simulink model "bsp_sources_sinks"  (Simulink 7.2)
settings: Solver=VariableStepDiscrete  StartTime=0.0  StopTime=1000.0  FixedStep=0.1  MaxStep=2.0  RelTol=1e-3
libraries: simulink x2

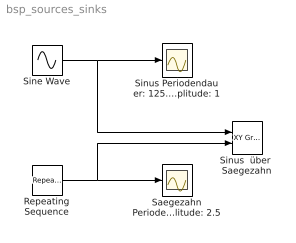
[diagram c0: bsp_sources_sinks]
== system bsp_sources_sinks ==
  Repeating Sequence : simulink/Sources/Repeating Sequence  SystemSampleTime=-1  rep_seq_t=[0:20:200]  rep_seq_y=[0:0.25:2.5 ]
  Saegezahn Periodendauer: 200s Amplitude: 2.5 : Scope
  Sine Wave : Sin  Frequency=0.05  SampleTime=0
  Sinus Periodendauer: 125.664s Amplitude: 1 : Scope
  Sinus  über  Saegezahn : simulink/Sinks/XY Graph  SystemSampleTime=-1  xmin=-1  xmax=1  ymin=0  ymax=2.5  st=-1
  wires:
  Repeating Sequence/1 -> Saegezahn Periodendauer: 200s Amplitude: 2.5/1, Sinus  über  Saegezahn/2
  Sine Wave/1 -> Sinus  über  Saegezahn/1, Sinus Periodendauer: 125.664s Amplitude: 1/1
